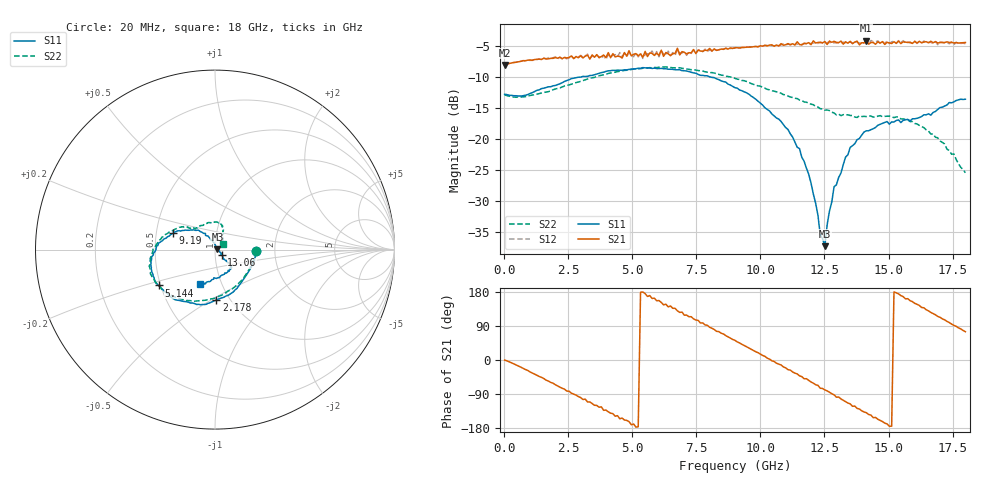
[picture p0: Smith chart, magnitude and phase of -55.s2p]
!Agilent Technologies,N5230A,US43500223,A.07.50.48
!Agilent N5230A: A.07.50.48
!Date: Monday, January 18, 2016 13:35:33
!Correction: S11(Full 2 Port(1,2))
!S21(Full 2 Port(1,2))
!S12(Full 2 Port(1,2))
!S22(Full 2 Port(1,2))
!S2P File: Measurements: S11, S21, S12, S22:
# Hz S  dB  R 50
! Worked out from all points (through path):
!   201 points, 20 MHz to 18 GHz, reference 50 ohm
!   highest |S21| = -4.05 dB at 14.13 GHz (marker M1); lowest = -8.0 dB at 20 MHz (marker M2)
!   group delay of S21, straight-line fit = 100 ps
!   lowest |S11| = -37.2 dB at 12.52 GHz (marker M3), VSWR 1.03, Z = 51.4 + j0.181 ohm
!   |S11| at or under -10 dB: start of sweep to 2.863 GHz; 8.119 GHz to end of sweep
!   |S22| runs from -25.4 to -8.3 dB; largest |S21 - S12| = 0.062
!   S11 on the Smith chart (normalised r, x): 20 MHz: 1.60, -0.03; 2.178 GHz: 0.87, -0.53; 5.144 GHz: 0.49, -0.23; 9.19 GHz: 0.61, +0.12; 13.06 GHz: 1.08, -0.07; 18 GHz: 0.79, -0.32
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2e7  -12.72 -2.1  -7.99 -0.1  -8.00 -0.2  -12.82 -1.9
9.19e8  -12.77 -46.9  -7.23 -27.5  -7.23 -27.9  -13.01 -43.9
2.1776e9  -11.03 -88.5  -6.74 -71.7  -6.74 -72.2  -11.70 -84.9
3.0766e9  -9.83 -108.6  -6.86 -104.1  -6.74 -104.0  -10.51 -107.1
4.2453e9  -8.86 -131.2  -6.17 -141.6  -6.39 -140.0  -9.22 -130.2
5.1443e9  -8.60 -147.5  -6.16 -177.2  -6.04 -178.5  -8.65 -144.2
6.0433e9  -8.57 -159.5  -6.43 157.0  -6.68 153.1  -8.36 -156.9
7.3918e9  -9.28 -175.8  -5.50 108.6  -5.61 109.4  -8.76 -172.0
9.01e9  -11.67 161.7  -5.21 51.8  -5.29 49.9  -10.16 169.7
9.1898e9  -12.04 158.3  -5.26 44.9  -5.26 43.1  -10.33 167.0
1.0808e10  -17.11 130.0  -4.56 -13.1  -4.78 -15.4  -12.56 148.2
1.15272e10  -21.48 117.0  -4.70 -41.8  -4.47 -43.5  -13.65 142.8
1.20666e10  -28.81 94.2  -4.11 -61.1  -4.45 -63.5  -14.40 140.0
1.25161e10  -37.22 7.4  -4.22 -78.8  -4.47 -80.6  -15.28 137.5
1.28757e10  -27.63 -31.3  -4.18 -91.8  -4.40 -94.1  -15.73 133.4
1.30555e10  -26.13 -40.3  -4.38 -97.8  -4.50 -100.9  -15.91 130.6
1.3505e10  -21.28 -46.0  -4.18 -115.7  -4.24 -118.6  -16.14 122.1
1.41343e10  -18.62 -44.9  -4.05 -139.1  -4.30 -141.7  -16.32 106.5
1.50333e10  -17.54 -51.1  -4.43 -174.8  -4.57 -176.4  -16.24 86.5
1.55727e10  -16.93 -58.7  -4.26 167.2  -4.08 163.7  -16.71 76.5
1.66515e10  -16.09 -92.3  -4.17 125.6  -4.35 119.9  -19.14 67.0
1.8e10  -13.52 -114.1  -4.37 74.7  -4.58 70.9  -25.38 35.8
